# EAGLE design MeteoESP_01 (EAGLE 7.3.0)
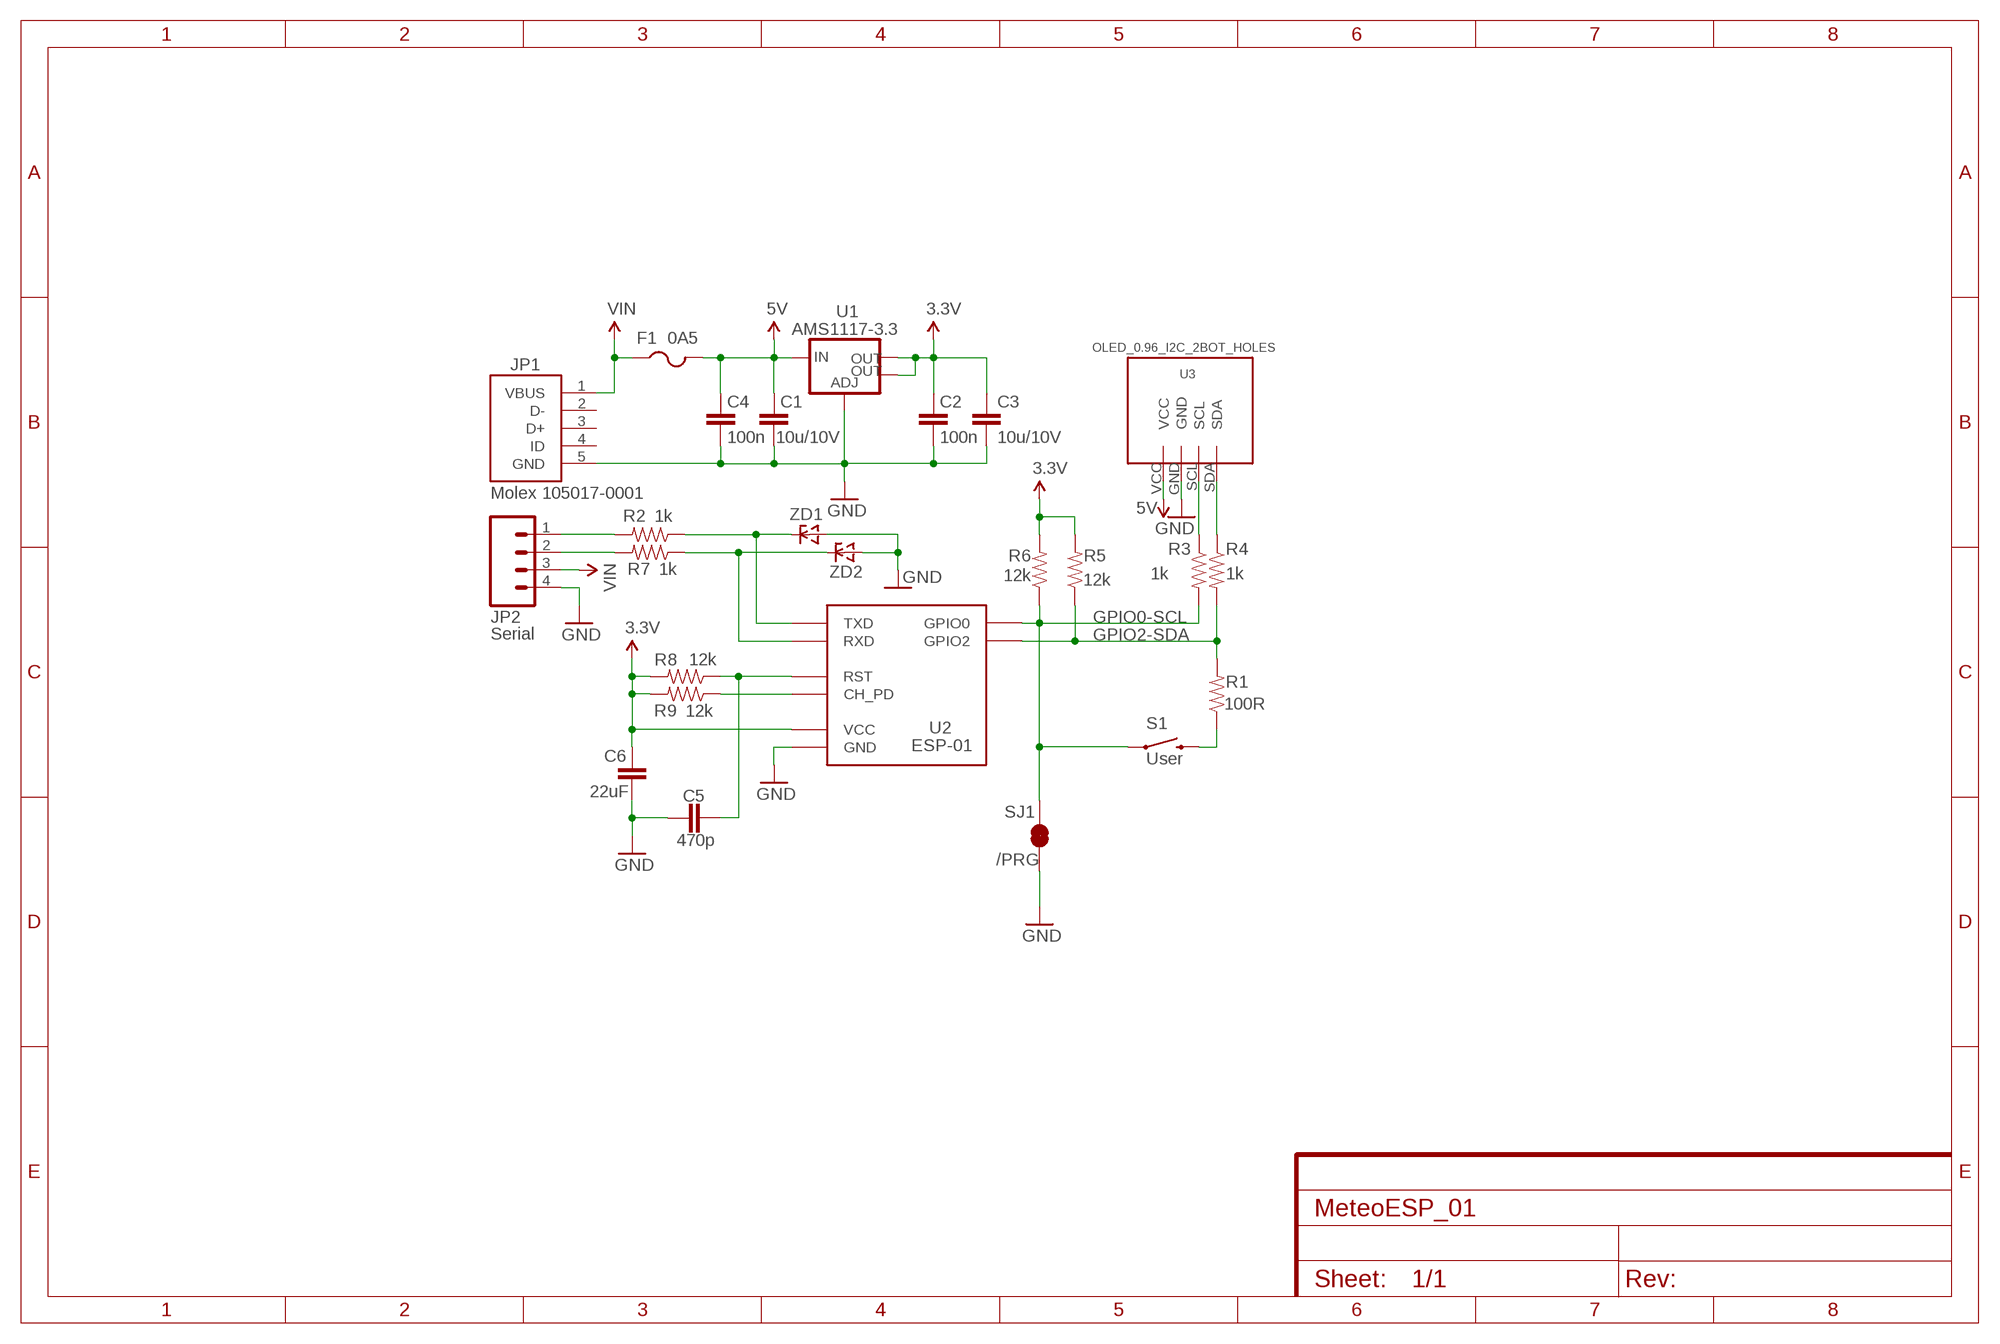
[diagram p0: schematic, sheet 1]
FRAME1 (FRAME-A4L): CNAME: MeteoESP; CREVISION: V1R0; DESIGNER: DonJuanito99

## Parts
C1  10u/10V  CAP1206  [1206]
C2  100n  CAP1206  [1206]
C3  10u/10V  CAP1206  [1206]
C4  100n  CAP1206  [1206]
C5  470p  CAP1206  [1206]
C6  22uF  CAP1206  [1206]
F1  0A5  PTCFUSE-1206  [R1206]
JP1  Molex 105017-0001  USB-CON-5PIN-105017-0001  [USB-MICRO-MOLEX-105017-0001]
JP2  Serial  M04POLAR_LOCK  [MOLEX-1X4_LOCK]
R1  100R  RESISTOR1206  [1206]
R2  1k  RESISTOR1206  [1206]
R3  1k  RESISTOR1206  [1206]
R4  1k  RESISTOR1206  [1206]
R5  12k  RESISTOR1206  [1206]
R6  12k  RESISTOR1206  [1206]
R7  1k  RESISTOR1206  [1206]
R8  12k  RESISTOR1206  [1206]
R9  12k  RESISTOR1206  [1206]
S1  User  SWITCH-MOMENTARY-2PTH  [TACTILE-PTH]
SJ1  /PRG  JUMPER-PAD-2-NC_BY_TRACE  [PAD-JUMPER-2-NC_BY_TRACE_YES_SILK]
U1  AMS1117-3.3  V_REG_LM1117SOT223  [SOT223]
U2  ESP-01  [ESP-01]
U3  OLED_0.96_I2C_2BOT_HOLES  OLED_0.96_I2C2BOTHOLES  [OLED_0.96_I2C_BOT2HOLES]
ZD1  ZENERSOD-123  [SOD-123]
ZD2  ZENERSOD-123  [SOD-123]

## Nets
3.3V: C2.1 C3.1 C6.1 R5.2 R6.2 R8.2 R9.2 U1.2(OUT) U1.4(OUT) U2.VCC
5V: C1.1 C4.1 F1.2 U1.3(IN) U3.VCC
CH_PD: R9.1 U2.CH_PD
GND: C1.2 C2.2 C3.2 C4.2 C5.2 C6.2 JP1.5(GND) JP2.4 SJ1.1 U1.1(ADJ) U2.GND U3.GND ZD1.A ZD2.A
GPIO0-SCL: R3.2 R6.1 S1.1 SJ1.2 U2.GPIO0
GPIO2-SDA: R1.2 R4.2 R5.1 U2.GPIO2
N$1: R7.1 U2.RX(RXD) ZD2.C
N$2: R2.1 U2.TX(TXD) ZD1.C
N$5: R1.1 S1.3
RESET: C5.1 R8.1 U2.RST
RX_E: JP2.2 R7.2
SCL: R3.1 U3.SCL
SDA: R4.1 U3.SDA
TX_E: JP2.1 R2.2
VIN: F1.1 JP1.1(VBUS) JP2.3
Unconnected: JP1.2(D-) JP1.3(D+) JP1.4(ID)

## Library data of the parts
C1-C5 = SparkFun-Passives:CAP: Capacitor
C6 = SparkFun-Capacitors:CAP: Capacitor
F1 = adafruit:PTCFUSE: PTC fuses, resettable thermistors
JP1 = Molex_JUAN:USB-CON-5PIN: Molex Micro USB 105017-0001 WARNING : Only for CNC production! The width of the contacts has been reduced to allow easy CNC routing...
JP2 = SparkFun-Connectors:M04: Header 4 Standard 4-pin 0.1" header. Use with straight break away headers (SKU : PRT-00116), right angle break away headers (PRT-00553), swiss pins (PRT-00743), machine pins (PRT-00117), and female headers (PRT-00115). Molex polarized connector foot print use with SKU : PRT-08231 with associated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
R1-R9 = SparkFun-Resistors:RESISTOR: Resistor
S1 = SparkFun-Electromechanical:SWITCH-MOMENTARY-2: Various NO switches- pushbuttons, reed, etc; PROD_ID: SWCH-08441
SJ1 = SparkFun-Passives:JUMPER-PAD-2-NC_BY_TRACE
U1 = SparkFun-PowerIC:V_REG_LM1117: Voltage Regulator LM1117 Standard adjustable voltage regulator but in SMD form. Spark Fun Electronics SKU : COM-00595; PROD_ID: VREG-08170
U2 = esp8266modules:ESP-01: ESP8266 Wifi Module ESP-01; DIMENSIONS: 14.3 x 24.8 mm; PINS: 8; PITCH: 0.1" / 2.54 mm
U3 = Oled_JUAN:OLED_0.96_I2C
ZD1 ZD2 = dp_devices:ZENER: Zener Diode SOD-323

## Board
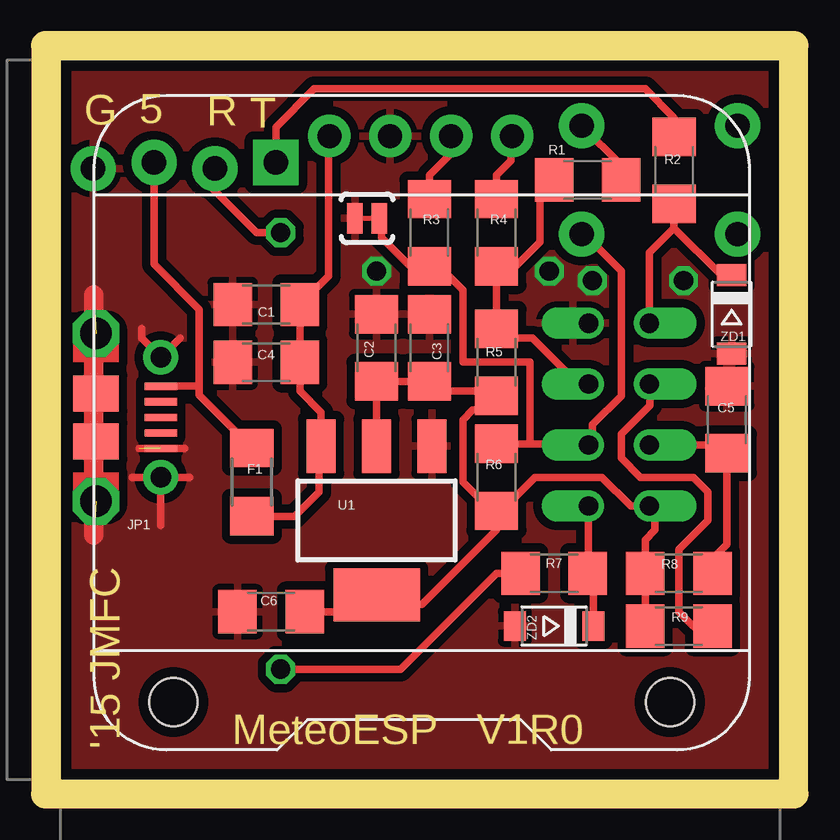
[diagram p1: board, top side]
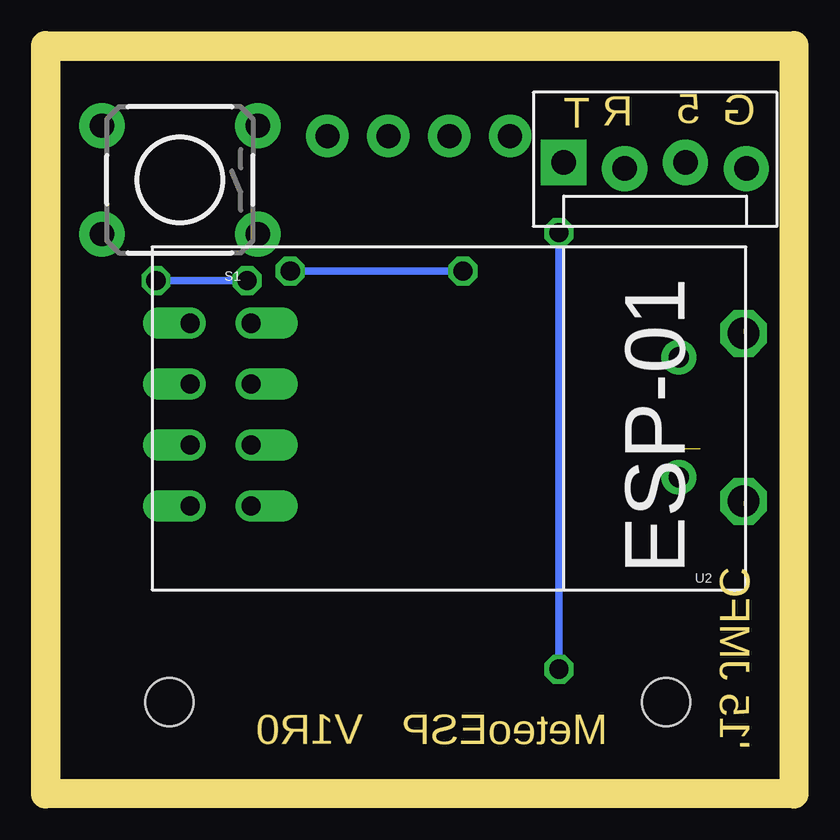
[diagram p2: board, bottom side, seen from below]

Size 30 x 30 mm. Coordinates in mm from the lower left corner, seen from the top.
Outline: 0,0 30,0 30,30 0,30 0,0
Copper layers (1*16): Top 0.035mm / dielectric 1.5mm / Bottom 0.035mm
Design rules "default": minimum track width 10mil, minimum drill 24mil, track to track 14mil, track to pad 14mil, pad to pad 14mil, via to via 14mil, smd to smd 14mil, copper to edge 18mil, drill to drill 8mil, minimum pad ring 10mil, minimum via ring 8mil, stop-mask expansion 4mil, vias tented up to drill 0mil, thermal gap 10mil
Milling: 4 lines

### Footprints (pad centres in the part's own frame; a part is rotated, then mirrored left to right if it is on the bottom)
1206 = smd 1.6 x 1.8: 1 -1.4,0; 2 1.4,0
R1206 = smd 1.6 x 1.803: 1 -1.422,0; 2 1.422,0
USB-MICRO-MOLEX-105017-0001 = smd 0.3 x 1.35: 1 1.2,0; 2 1.85,0; 3 2.5,0; 4 3.15,0; 5 3.8,0 | drill 0.85 pad 1.45: P$1 0,0; P$2 5,0 | smd 1.5 x 1.9: P$3 3.5,-2.7; P$4 1.5,-2.7
MOLEX-1X4_LOCK = drill 1.016 pad 1.88 square: 1 0,0.127 | drill 1.016 pad 1.88: 2 2.54,-0.127; 3 5.08,0.127; 4 7.62,-0.127
TACTILE-PTH = drill 1.016 pad 1.88: 1 -3.251,2.261; 2 3.251,2.261; 3 -3.251,-2.261; 4 3.251,-2.261
PAD-JUMPER-2-NC_BY_TRACE_YES_SILK = smd 0.635 x 1.27: 1 -0.508,0; 2 0.508,0
SOT223 = smd 1.219 x 2.235: 1 -2.311,-3.099; 2 0,-3.099; 3 2.311,-3.099 | smd 3.6 x 2.2: 4 0,3.099
ESP-01 = drill 0.8 offset: CH_PD -1.285,-8.178; GND -3.825,-5.638; GPIO0 1.255,-5.638; GPIO2 -1.285,-5.638; RST 1.255,-8.178; RX 3.795,-5.638; TX -3.825,-8.178; VCC 3.795,-8.178
OLED_0.96_I2C_BOT2HOLES = drill 1 pad 1.778: GND -1.63,11.63; SCL 0.91,11.63; SDA 3.45,11.63; VCC -4.17,11.63 | hole 2: -10.67,-11.97; 10.03,-11.97
SOD-123 = smd 0.91 x 1.22: A 1.635,0; C -1.635,0

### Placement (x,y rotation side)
C1  8.6,19.8 180 top
C2  13.2,18 90 top
C3  15.4,18 90 top
C4  8.6,17.4 180 top
C5  27.8,15 90 top
C6  8.8,7 180 top
F1  8,12.4 270 top
JP1  4.2,17.6 270 top
JP2  9,25.6 0 bottom
R1  22,25 180 top
R2  25.6,25.4 90 top
R3  15.4,22.8 270 top
R4  18.2,22.8 270 top
R5  18.2,17.4 270 top
R6  18.2,12.6 270 top
R7  20.6,8.6 180 top
R8  25.8,8.6 180 top
R9  25.8,6.4 180 top
S1  25,25 180 bottom
SJ1  12.8,23.4 0 top
U1  13.2,10.8 180 top
U2  16.4,15.2 270 bottom
U3  15.4,15.2 0 top
ZD1  28,19.4 270 top
ZD2  20.6,6.4 180 top

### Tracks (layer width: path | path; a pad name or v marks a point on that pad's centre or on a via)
3.3V
  Top 0.305: U1.2 C2.1 C3.1 15.8,16.2 18.2,16.2 R5.2 17.6,15.4 17.2,15.4 16.8,15 16.8,12.4 18,11.2 R6.2 | R6.2 18.4,11.2 19.8,12.6 22.6,12.6 23.8,11.4 24.6,11.4 24.59,11.4 U2.VCC 24.8,11.18 24.8,10.4 24.4,10 R8.2 R9.2 | R6.2 18.2,10.4 15.1,7.3 13.6,7.3 13.3,7.6 13.2,7.6 | 13.2,7.6 U1.4 | C6.1 12.6,7 13.2,7.6
5V
  Top 0.305: F1.2 9.78,10.98 10.8,12 10.8,13.81 U1.3 10.89,15.31 10,16.2 10,17.2 C4.1 C1.1 11.2,21 11.2,26.8 U3.VCC
CH_PD
  Top 0.305: R9.1 27,5.8 25.8,7 25.8,9.2 25.8,9.6 27,10.8 27,11 27,12 26.4,12.6 24.2,12.6 23.4,13.4 23.4,14.4 24.6,15.6 24.6,16.4 24.58,16.42 U2.CH_PD
GND  (via drill 0.8, 1.3)  (3 unrouted)
  Top 0.305: 4.2,10.6 4.2,12.6 | 3.4,18.8 3.4,18.4 4.2,17.6 5,18.4 | 4.2,12.6 5.4,12.6 | 4.2,12.6 3,12.6 | 3.3,13.8 5.2,13.8
  Top 0.813: 1.4,10.2 1.4,20.2
  Bottom 0.305: v22.2,20.8 v26,20.8 | v13.2,21.2 v20.4,21.2
  other vias: 1.5,11.6 1.5,18.6
  pour Top: 0.2,29.8 29.8,29.8 29.8,0.2 0.2,0.2
GPIO0-SCL
  Top 0.305: 19.6,14 R6.1 | 19.6,14 22.04,14 U2.GPIO0 22.2,14.11 22.2,14.8 23.4,16 23.4,17 23.4,21.2 22,22.6 21.8,22.8 S1.1 | 19.6,14 19.6,17.4 16.8,17.4 16.8,18 16.8,20.4 15.8,21.4 R3.2 14.6,21.4 13.4,22.6 13.4,23.4 SJ1.2
GPIO2-SDA
  Top 0.305: U2.GPIO2 22,16.45 22,16.4 21.7,16.4 19.7,18.4 18.2,18.4 R5.1 R4.2 19,21.4 20,22.4 20,24.4 R1.2
N$1
  Top 0.305: ZD2.C 22.23,8.37 R7.1 22.04,8.64 U2.RX
N$2
  Top 0.305: U2.TX 24.58,21.98 25.6,23 | 25.6,23 25.6,23.8 R2.1 | ZD1.C 27.57,21.04 25.6,23
N$5
  Top 0.305: S1.3 23.4,25.61 R1.1
RESET
  Top 0.305: R8.1 27.2,9.2 27.8,9.8 C5.1 27.66,13.95 U2.RST
RX_E  (via drill 0.8)
  Top 0.305: v9.2,4.6 14.2,4.6 18.2,8.6 R7.2 | v9.2,22.8 8.2,22.8 6.4,24.6 6.4,25.41 JP2.2
  Bottom 0.305: v9.2,22.8 v9.2,4.6
SCL
  Top 0.305: R3.1 15.4,25.2 16.4,26.2 16.4,26.74 U3.SCL
SDA
  Top 0.305: R4.1 18.2,25.2 18.8,25.8 18.8,26.78 U3.SDA
TX_E
  Top 0.305: R2.2 25.6,27.6 24.4,28.8 10.6,28.8 9,27.2 JP2.1
VIN
  Top 0.305: 8,14.2 F1.1 5.8,16.02 5.8,16.4 | 5.8,16.4 5.8,19.6 3.92,21.48 JP2.3 | JP1.1 5.8,16.4

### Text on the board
Milling: G | 5 | R | T | '15 JMFC | MeteoESP | V1R0

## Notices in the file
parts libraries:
SparkFun-PowerIC: Licensing: Creative Commons ShareAlike 4.0 International - https://creativecommons.org/licenses/by-sa/4.0
